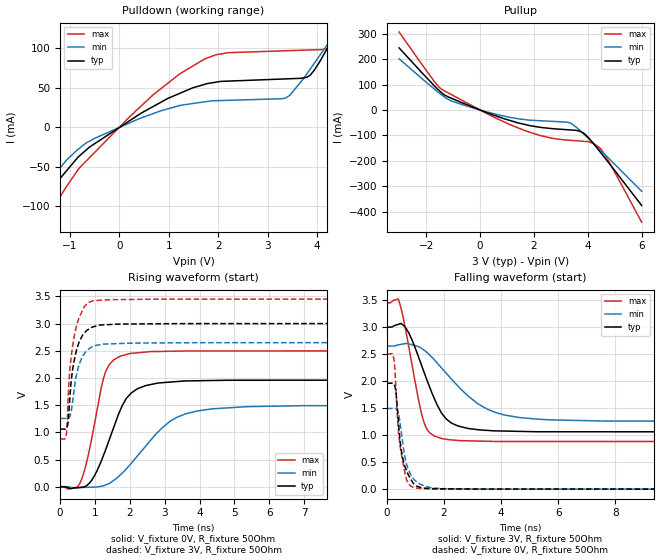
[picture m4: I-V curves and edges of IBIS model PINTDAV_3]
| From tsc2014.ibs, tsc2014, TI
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|   3V PINTDAV Model
[Model] PINTDAV_3
Model_type Output
Polarity   Non-Inverting
Enable   Active-Low
Vmeas = 1.5
Vref = 1.5
Cref = 15pF
Rref = 50
|   typ   min   max
|   C_comp average
C_comp   1.6054806E-11   8.8879840E-12   5.1098196E-11
|   C_comp high output
|C_comp   6.1933510e-12   6.1927020e-12   7.0694780e-12
|   C_comp low output
|C_comp   2.5916910e-11   1.0706490e-11   9.6003040e-11
|Where nom PVT is NOM Process, 3V,27C
|   Fast PVT is Strong Process, 3.45V, -40C
|   Slow PVT is Weak Process, 2.65V, 85C
[Voltage Range]   3   2.65   3.45
[Temperature Range]   27   85   -40
[Pullup Reference]   3   2.65   3.45
[Pulldown Reference]   0   0   0
[Power Clamp Reference]   3   2.65   3.45
[GND Clamp Reference]   0   0   0
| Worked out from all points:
|   slope of the pulldown table from 0 to 0.45 V, typ, clamps not added: 24.3 ohm
|   slope of the pullup table from 0 to 0.45 V, typ, clamps not added: 24.6 ohm
|   falling waveform, V_fixture 3V, R_fixture 50Ohm: 20-80 % time 882ps typ, 1.64ns min, 556ps max; typ from 3 V to 1.06 V
|   rising waveform, V_fixture 0V, R_fixture 50Ohm: 20-80 % time 723ps typ, 1.28ns min, 470ps max; typ from 0 V to 1.96 V
|   rising waveform, V_fixture 3V, R_fixture 50Ohm: 20-80 % time 259ps typ, 275ps min, 246ps max; typ from 1.06 V to 3 V
|   falling waveform, V_fixture 0V, R_fixture 50Ohm: 20-80 % time 292ps typ, 338ps min, 255ps max; typ from 1.96 V to 0 V
[Pulldown]
|   Voltage   I(typ)   I(min)   I(max)
-3V       -288.9mA   -229.2mA   -403.1mA
-2.014V   -157.4mA   -128.3mA   -211.3mA
-1.738V   -122.5mA   -100.9mA   -159.3mA
-1.557V   -99.6mA    -83.37mA   -128mA
-670.9mV  -28.88mA   -20.03mA   -42.85mA
681.2mV   26.09mA    17.1mA     40.9mA
1.735V    54.44mA    32.16mA    86.62mA
3.375V    61.18mA    37.23mA    96.86mA
3.862V    65.92mA    73.59mA    97.88mA
4.464V    128.2mA    128mA      109.6mA
4.87V     175.5mA    165.9mA    166mA
5.991V    310.6mA    273.3mA    342.3mA
[Pullup]
|   Voltage   I(typ)   I(min)   I(max)
-3V       243.9mA    201.2mA    306.3mA
-1.73V    99.06mA    85.73mA    116.9mA
-1.375V   63.24mA    55.64mA    78.51mA
-1.044V   45.52mA    34.92mA    59.57mA
182.4mV   -7.289mA   -5.517mA   -10.01mA
1.666V    -56.81mA   -37.79mA   -80.99mA
2.697V    -73.25mA   -44.65mA   -111.5mA
3.303V    -77.93mA   -49.4mA    -118.7mA
3.838V    -90.81mA   -93.4mA    -122.8mA
4.398V    -157.1mA   -150.9mA   -144.9mA
4.764V    -206.5mA   -189mA     -200.3mA
5.991V    -374.8mA   -319mA     -440.7mA
[Ramp]
R_load = 50
|   typ   min   max
dV/dt_r   1.17612/7.17238e-010  0.896321/1.28248e-009   1.49874/4.67518e-010
dV/dt_f   1.16427/8.77952e-010  0.837293/1.62697e-009   1.54181/5.54059e-010
[Falling Waveform]
V_fixture = 3V
V_fixture_min = 2.65V
V_fixture_max = 3.45V
R_fixture = 50Ohm
C_fixture = 0F
|   Time   V(typ)   V(min)   V(max)
0s        3V         2.65V      3.45V
396.2ps   3.052V     2.672V     3.513V
756.7ps   2.9V       2.691V     2.653V
1.277ns   2.197V     2.582V     1.27V
1.488ns   1.899V     2.486V     1.049V
1.882ns   1.437V     2.262V     942.5mV
2.256ns   1.225V     2.039V     911.7mV
3.198ns   1.101V     1.578V     890.8mV
4.677ns   1.07V      1.325V     882.8mV
20ns      1.06V      1.255V     880.3mV
[Rising Waveform]
V_fixture = 0V
V_fixture_min = 0V
V_fixture_max = 0V
R_fixture = 50Ohm
C_fixture = 0F
|   Time   V(typ)   V(min)   V(max)
0s        104.7nV    200.9nV    48.99nV
516.8ps   -14.91mV   -21.52mV   12.64mV
683.3ps   -4.613mV   -12.13mV   265.6mV
908.5ps   122.6mV    -8.39mV    897.7mV
1.31ns    688.9mV    33.52mV    2.123V
1.684ns   1.349V     193.3mV    2.386V
1.976ns   1.679V     383.7mV    2.445V
3.17ns    1.925V     1.209V     2.49V
4.394ns   1.953V     1.433V     2.496V
20ns      1.96V      1.494V     2.498V
[Rising Waveform]
V_fixture = 3V
V_fixture_min = 2.65V
V_fixture_max = 3.45V
R_fixture = 50Ohm
C_fixture = 0F
|   Time   V(typ)   V(min)   V(max)
0s        1.06V      1.255V     880.3mV
176.5ps   1.071V     1.254V     957.9mV
197.5ps   1.097V     1.254V     1.135V
228.8ps   1.196V     1.256V     1.62V
282.7ps   1.664V     1.3V       2.175V
347.5ps   2.104V     1.517V     2.536V
452.6ps   2.466V     2.006V     2.916V
654.9ps   2.795V     2.409V     3.261V
939ps     2.938V     2.576V     3.42V
20ns      3V         2.65V      3.45V
[Falling Waveform]
|Gnd
V_fixture = 0V
V_fixture_min = 0V
V_fixture_max = 0V
R_fixture = 50Ohm
C_fixture = 0F
|   Time   V(typ)   V(min)   V(max)
0s        1.96V      1.494V     2.498V
246.6ps   1.942V     1.495V     2.394V
310.3ps   1.807V     1.491V     1.87V
405.5ps   1.209V     1.389V     1.036V
478.9ps   798.6mV    1.139V     724.3mV
625.7ps   423.5mV    602.7mV    305.2mV
747.8ps   264.3mV    365.5mV    102.4mV
965.7ps   88.25mV    169.2mV    24.51mV
2.106ns   5.324mV    6.957mV    4.065mV
20ns      80.01nV    142nV      32.85nV
